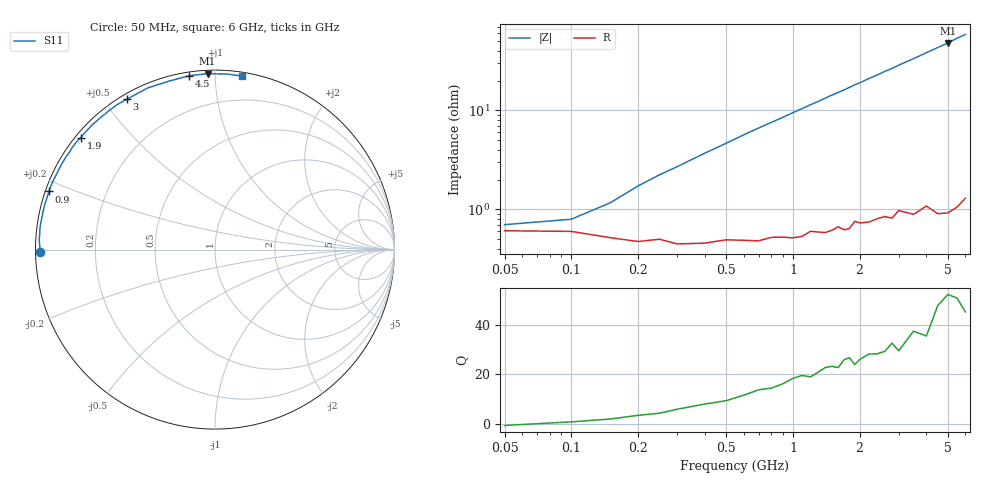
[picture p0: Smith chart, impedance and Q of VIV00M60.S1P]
! Infineon Technologies  Discrete & RF Semiconductors
! BB 804
! Si Tuning Diode in SOT23
! VR =
! S-Parameters:  July  1999
# GHz  S  MA  R  50
!  f  S11
! GHz  MAG  ANG
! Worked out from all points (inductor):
!   34 points, 50 MHz to 6 GHz, reference 50 ohm
!   read as one part to ground: L = 1.39 nH near 200 MHz
!   highest Q = 50.7 at 5 GHz (marker M1), where L = 1.53 nH
!   S11 on the Smith chart (normalised r, x): 50 MHz: 0.01, -0.01; 900 MHz: 0.01, +0.17; 1.9 GHz: 0.02, +0.36; 3 GHz: 0.02, +0.57; 4.5 GHz: 0.02, +0.86; 6 GHz: 0.03, +1.17
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0.05  0.9759 -179.2
0.1  0.9763 178.8
0.2  0.9812 176.2
0.25  0.9802 175.0
0.3  0.9823 173.9
0.4  0.982 171.6
0.7  0.9812 164.9
0.8  0.9798 162.8
0.9  0.9798 160.7
1.1  0.9797 156.4
1.3  0.9779 152.3
1.5  0.9775 148.1
1.6  0.9758 146.2
1.7  0.9777 144.3
1.8  0.9773 142.2
1.9  0.9736 140.1
2  0.9747 138.4
2.2  0.975 134.5
2.4  0.9736 131.0
2.6  0.9732 127.2
2.8  0.9748 124.0
3  0.9711 120.4
3.5  0.9756 112.6
4  0.9731 105.1
4.5  0.9794 98.4
5  0.981 92.4
5.5  0.9805 86.0
6  0.9783 81.0
